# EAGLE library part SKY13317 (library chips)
20-6000 MHZ SP3T RF Switch
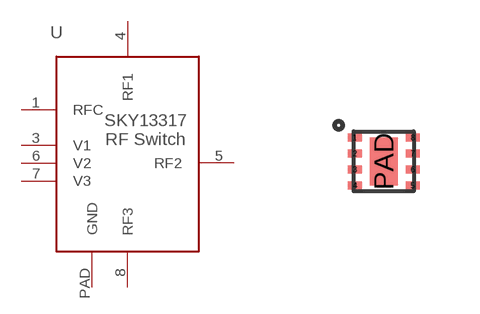
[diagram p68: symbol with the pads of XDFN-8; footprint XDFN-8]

Designator prefix U

## SKY13317 (DIGIKEY: 863-1056-1-ND; MANUFACTURER: Skworks Solutions; MPN: SKY13317-373LF)  [XDFN-8]
1  RFC
3  V1
4  RF1
5  RF2
6  V2
7  V3
8  RF3
PAD  GND

## Footprint XDFN-8 (pad centres in mm)
smd 0.35 x 0.2: 1 0.025,1.35; 2 0.025,0.95; 3 0.025,0.55; 4 0.025,0.15; 5 1.475,0.15; 6 1.475,0.55; 7 1.475,0.95; 8 1.475,1.35
smd 0.7 x 1.2: PAD 0.75,0.75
